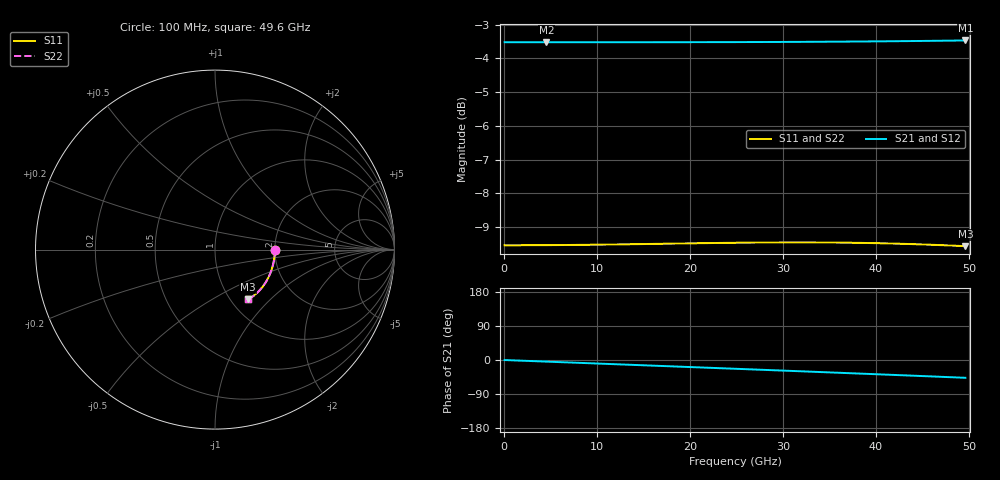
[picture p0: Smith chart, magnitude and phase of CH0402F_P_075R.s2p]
# GHz S RI R 75
! S-Parameters data
! Freq  reS11  imS11  reS21  imS21  reS12  imS12  reS22  imS22
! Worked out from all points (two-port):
!   100 points, 100 MHz to 49.6 GHz, reference 75 ohm
!   highest |S21| = -3.47 dB at 49.6 GHz (marker M1); lowest = -3.5 dB at 4.6 GHz (marker M2)
!   |S21| within 3 dB of the highest: start of sweep to end of sweep
!   lowest |S11| = -9.6 dB at 49.6 GHz (marker M3), VSWR 2.00, Z = 89.8 - j55.9 ohm
!   |S11| at or under -10 dB: nowhere
!   |S22| runs from -9.6 to -9.5 dB; largest |S21 - S12| = 0
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0.1  0.3333 -0.000806  0.6667 -0.00108  0.6667 -0.00108  0.3333 -0.000806
2.1  0.3329 -0.0169  0.6663 -0.0226  0.6663 -0.0226  0.3329 -0.0169
4.6  0.3314 -0.037  0.6648 -0.0496  0.6648 -0.0496  0.3314 -0.037
6.6  0.3294 -0.0529  0.6629 -0.0711  0.6629 -0.0711  0.3294 -0.0529
8.6  0.3267 -0.0686  0.6602 -0.0925  0.6602 -0.0925  0.3267 -0.0686
10.6  0.3234 -0.084  0.6569 -0.1138  0.6569 -0.1138  0.3234 -0.084
12.6  0.3193 -0.0991  0.6529 -0.1351  0.6529 -0.1351  0.3193 -0.0991
16.6  0.3095 -0.1282  0.6428 -0.1772  0.6428 -0.1772  0.3095 -0.1282
20.6  0.2974 -0.1555  0.6299 -0.2187  0.6299 -0.2187  0.2974 -0.1555
22.6  0.2907 -0.1684  0.6225 -0.2391  0.6225 -0.2391  0.2907 -0.1684
25.1  0.2817 -0.1836  0.6123 -0.2644  0.6123 -0.2644  0.2817 -0.1836
29.1  0.2662 -0.2059  0.5939 -0.3042  0.5939 -0.3042  0.2662 -0.2059
31.1  0.2581 -0.2161  0.5837 -0.3237  0.5837 -0.3237  0.2581 -0.2161
33.1  0.2498 -0.2256  0.5728 -0.343  0.5728 -0.343  0.2498 -0.2256
35.1  0.2414 -0.2344  0.5613 -0.362  0.5613 -0.362  0.2414 -0.2344
37.1  0.233 -0.2424  0.5491 -0.3807  0.5491 -0.3807  0.233 -0.2424
39.1  0.2246 -0.2498  0.5362 -0.3991  0.5362 -0.3991  0.2246 -0.2498
41.6  0.2143 -0.2579  0.5192 -0.4217  0.5192 -0.4217  0.2143 -0.2579
43.6  0.2062 -0.2637  0.5049 -0.4394  0.5049 -0.4394  0.2062 -0.2637
45.6  0.1984 -0.2688  0.4898 -0.4568  0.4898 -0.4568  0.1984 -0.2688
47.6  0.1908 -0.2732  0.4741 -0.4737  0.4741 -0.4737  0.1908 -0.2732
49.6  0.1837 -0.2769  0.4576 -0.4903  0.4576 -0.4903  0.1837 -0.2769
